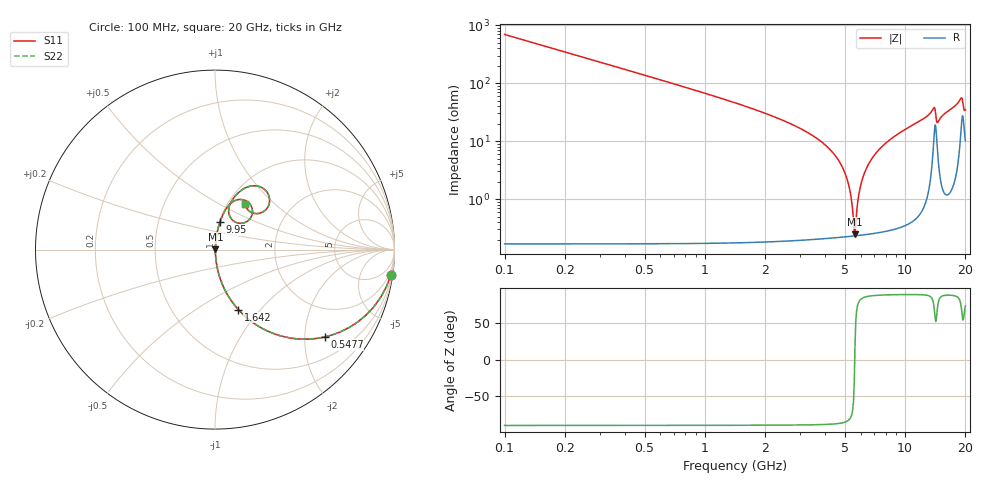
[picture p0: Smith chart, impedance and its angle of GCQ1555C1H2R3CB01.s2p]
!Murata Part Number: GCQ1555C1H2R3CB01
!These Parameters are Measured in Series Mode Connection
!Data Generated on Mar 13, 2026
!  o--ll--o
!Port1  Port2
!  o------o
!Operation Temp=25[degC], DC Bias Voltage=0[V]
!Freq. Start=100[MHz] Stop=20[GHz] 401[Steps]
# Hz S RI R 50
!Freq.(Hz) S11(Real) S11(Imag) S21(Real) S21(Imag) S12(Real) S12(Imag) S22(Real) S22(Imag)
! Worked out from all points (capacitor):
!   401 points, 100 MHz to 20 GHz, reference 50 ohm
!   read as one part in series: C = 2.3 pF near 199.5 MHz
!   lowest |Z| = 246 mohm at 5.622 GHz (marker M1)
!   series resonance near 5.604 GHz, so ESL is about 350 pH
!   S11 on the Smith chart (normalised r, x): 100 MHz: 1, -14; 547.8 MHz: 1.00, -2.50; 1.642 GHz: 1.00, -0.77; 9.95 GHz: 1.01, +0.31; 20 GHz: 1.20, +0.67
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1e8  0.9795 -0.1416  0.0205 0.1416  0.0205 0.1416  0.9795 -0.1416
2.99e8  0.8417 -0.3646  0.1583 0.3646  0.1583 0.3646  0.8417 -0.3646
5.4775e8  0.6101 -0.487  0.3899 0.487  0.3899 0.487  0.6101 -0.487
1.04525e9  0.2906 -0.4527  0.7094 0.4527  0.7094 0.4527  0.2906 -0.4527
1.64225e9  0.1305 -0.3345  0.8695 0.3345  0.8695 0.3345  0.1305 -0.3345
3.43325e9  0.0176 -0.1239  0.9824 0.1239  0.9824 0.1239  0.0176 -0.1239
4.92575e9  0.00324 -0.032  0.9968 0.032  0.9968 0.032  0.00324 -0.032
5.274e9  0.00249 -0.0151  0.9975 0.0151  0.9975 0.0151  0.00249 -0.0151
5.52275e9  0.00231 -0.00363  0.9977 0.00363  0.9977 0.00363  0.00231 -0.00363
5.62225e9  0.00232 0.00081  0.9977 -0.00081  0.9977 -0.00081  0.00232 0.00081
6.02025e9  0.0027 0.0179  0.9973 -0.0179  0.9973 -0.0179  0.0027 0.0179
6.7665e9  0.00475 0.0473  0.9952 -0.0473  0.9952 -0.0473  0.00475 0.0473
8.01025e9  0.0112 0.0913  0.9888 -0.0913  0.9888 -0.0913  0.0112 0.0913
9.9505e9  0.0273 0.1525  0.9727 -0.1525  0.9727 -0.1525  0.0273 0.1525
1.005e10  0.0284 0.1555  0.9716 -0.1555  0.9716 -0.1555  0.0284 0.1555
1.338325e10  0.1015 0.2681  0.8985 -0.2681  0.8985 -0.2681  0.1015 0.2681
1.398025e10  0.197 0.251  0.803 -0.251  0.803 -0.251  0.197 0.251
1.447775e10  0.0997 0.1624  0.9003 -0.1624  0.9003 -0.1624  0.0997 0.1624
1.67165e10  0.1158 0.3021  0.8842 -0.3021  0.8842 -0.3021  0.1158 0.3021
1.895525e10  0.2727 0.3379  0.7273 -0.3379  0.7273 -0.3379  0.2727 0.3379
1.95025e10  0.2506 0.2028  0.7494 -0.2028  0.7494 -0.2028  0.2506 0.2028
2e10  0.1684 0.2522  0.8316 -0.2522  0.8316 -0.2522  0.1684 0.2522
